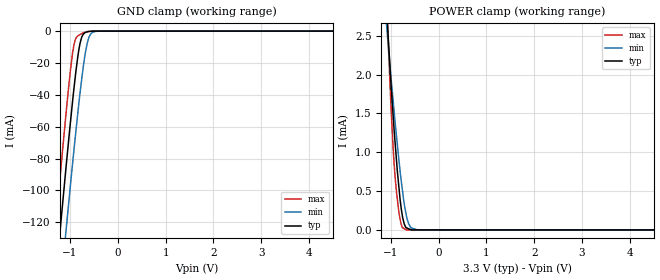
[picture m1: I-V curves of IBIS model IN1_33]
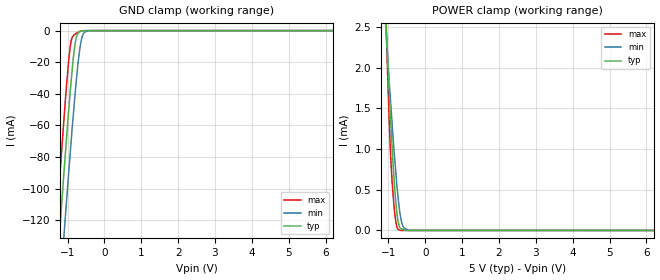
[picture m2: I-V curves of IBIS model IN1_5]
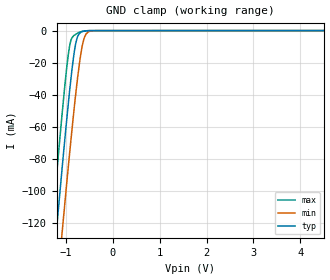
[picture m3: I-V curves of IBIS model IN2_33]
|Texas Instruments Incorporated
|Power Line Communications Analog Front End
| Marketing part#   Digital Voltage Range   Package-type   #pins
|AFE030AIRGZR   2.7 to 5.5 V   VQFN   48
|AFE030AIRGZT   2.7 to 5.5 V   VQFN   48
[IBIS Ver]   4.0
[File name]   afe030.ibs
[File Rev]   1.0
[Date]   11/12/2010
[Source]   Texas Instruments Incorporated.
   Analog-eLab, HPA
   12500 TI Blvd
   Dallas, TX -75243
   For Support e-mail: elab_ibis@list.ti.com
[Notes]   Revision History:
   1.0: 11/12/2010
   - Initial version of the model
   - Initial Model generated from simulations in TISPICED
   - Model names with a trailing _33 contains the model for
   3.3V (3V and 3.6V).
   _ Model names with trailing _5 contains
   the model for 5V (4.5V and 5.5V) operation.
   - Model not matched to measurements
   - C_comp although listed in numerical order of value are
   obtained from varying PVT conditions. For PVT conditions
   for each specific value refer the buffer description under
   respective [Model]. IBIS model user is responsible for using
   appropriate C_comp to simulate for Signal Integrity.
   - Combined nonmonitonicity of OUT_33 and OUT_5 pulldown and
   pullup data is inherent to buffers as seen in simulations
[Disclaimer]
 This product is designed as an aid for customers of Texas Instruments.
 No warranties, either expressed or implied, with respect to this third
 party software (if any) or with respect to its fitness for any
 particular purpose is claimed by Texas Instruments or the author. The
 software (if any) is provided solely on an "as is" basis. The entire
 risk as to its quality and performance is with the customer
[Copyright] (C) Copyright 2009 Texas Instruments Incorporated.
   All rights reserved.
|   AFE031
[Component]   AFE031
[Manufacturer] TI
[Package]   | 48 QFN - RGZ package
| variable   typ   min   max
R_pkg  4.37953E-02   3.97800E-02   4.78600E-02
L_pkg  1.49490E+00nH 1.30880E+00nH 1.70496E+00nH
C_pkg  3.20541E-01pF 3.01690E-01pF 3.38680E-01pF
|-------------------------PIN------------------------------------------------
[Pin] signal_name  model_name  R_pin  L_pin C_pin
1  DGnd   GND   0.04794  1.70441nH  0.32378pF
2  DVdd   POWER  0.04526  1.58988nH  0.33894pF
3  SCLK   IN1   0.04305  1.48606nH  0.32786pF
4  DIN   IN1   0.04124  1.40172nH  0.31704pF
5  DOUT   OUT1   0.04012  1.34655nH  0.30872pF
6  CS   IN1   0.03982  1.32719nH  0.30169pF
7  DAC   IN1   0.04021  1.33885nH  0.30263pF
8  SD   IN1   0.04128  1.38204nH  0.30973pF
9  INT   OUT2   0.04165  1.41439nH  0.31629pF
10 TSense   TERM   0.04363  1.50387nH  0.32778pF
11 AVdd1   POWER  0.04489  1.57822nH  0.33524pF
12 AGnd1   GND   0.04663  1.66363nH  0.31950pF
13 Tx_PGA_In   TERM   0.04786  1.70496nH  0.31944pF
14 Tx_PGA_Out   TERM   0.04650  1.63128nH  0.33542pF
15 Tx_F_In1   TERM   0.04547  1.56285nH  0.32756pF
16 Tx_F_In2   TERM   0.04465  1.50749nH  0.31973pF
17 Tx_F_Out   TERM   0.04404  1.46688nH  0.31329pF
18 PA_In   TERM   0.04373  1.44633nH  0.30627pF
19 C1   TERM   0.04363  1.44263nH  0.30600pF
20 Rx_PGA2_Out  TERM   0.04374  1.45568nH  0.31243pF
21 Rx_PGA2_In   TERM   0.04415  1.48905nH  0.31836pF
22 Rx_F_Out   TERM   0.04479  1.53774nH  0.32624pF
23 Rx_C2   TERM   0.04597  1.60959nH  0.33499pF
24 Rx_C1   TERM   0.04761  1.69090nH  0.31944pF
25 Rx_F_In   TERM   0.04666  1.64938nH  0.32310pF
26 Rx_PGA1_Out  TERM   0.04436  1.54523nH  0.33868pF
27 Rx_PGA1_In   TERM   0.04253  1.45348nH  0.32802pF
28 C2   TERM   0.04110  1.38100nH  0.31750pF
29 AGnd2   GND   0.04027  1.33462nH  0.30931pF
30 AVdd2   POWER  0.03989  1.31213nH  0.30236pF
31 E_Rx_Out   TERM   0.03978  1.30880nH  0.30230pF
32 E_Rx_In   TERM   0.04003  1.32739nH  0.30911pF
33 E_Tx_Out   OUT1   0.04080  1.37171nH  0.31662pF
34 E_Tx_In   IN2   0.04200  1.43702nH  0.32606pF
35 E_Tx_Clk   IN2   0.04357  1.52060nH  0.33618pF
36 ZC_Out2   TERM   0.04571  1.61986nH  0.32130pF
37 ZC_Out1   TERM   0.04717  1.66751nH  0.32302pF
38 ZC_In2   IN3   0.04609  1.60204nH  0.33837pF
39 ZC_In1   IN3   0.04599  1.56391nH  0.33217pF
40 PA_Gnd2   GND   0.04479  1.49878nH  0.32458pF
41 PA_Gnd1   GND   0.04400  1.45436nH  0.32078pF
42 PA_Out2   TERM   0.04316  1.41904nH  0.31296pF
43 PA_Out1   TERM   0.04316  1.41958nH  0.31068pF
44 PA_Vs2   TERM   0.04358  1.44390nH  0.31762pF
45 PA_Vs1   TERM   0.04427  1.48688nH  0.32403pF
46 PA_Iset   TERM   0.04563  1.55774nH  0.33228pF
47 Tx_Flag   OUT2   0.04599  1.60396nH  0.33861pF
48 Rx_Flag   OUT2   0.04709  1.67076nH  0.32210pF
|   Model Selectors
[Model Selector]  IN1
IN1_33  3.3V digital input
IN1_5   5V digital input
|NOTES   Model IN1 split into two Models IN1_33 and IN1_5
|   to accomodate vast voltage range of 2.7V - 5.5V
|   IN1_33 operates in voltage range of 3 - 3.3 - 3.6
|   IN1_5 operates in voltage range of 4.5 - 5 - 5.5
|   The max pin frequency for Model IN1 is 20MHz.Also the
|   voltage range and frequency is referenced with datasheet.
[Model Selector]  IN2
IN2_33  3.3V digital input
IN2_5   5V digital input
|NOTES   Model IN2 split into two Models IN2_33 and IN2_5
|   to accomodate vast voltage range of 2.7V - 5.5V
|   IN2_33 operates in voltage range of 3 - 3.3 - 3.6
|   IN2_5 operates in voltage range of 4.5 - 5 - 5.5
|   The max pin frequency for Model IN2 is 20MHz.Also the
|   voltage range and frequency is referenced with datasheet.
[Model Selector]  IN3
IN3_33  3.3V digital input
IN3_5   5V digital input
|NOTES   Model IN1 split into two Models IN3_33 and IN3_5
|   to accomodate vast voltage range of 2.7V - 5.5V
|   IN3_33 operates in voltage range of 3 - 3.3 - 3.6
|   IN3_5 operates in voltage range of 4.5 - 5 - 5.5
|   The max pin frequency for Model IN3 is 20MHz.Also the
|   voltage range and frequency is referenced with datasheet.
[Model Selector]  OUT1
OUT1_33 3.3V digital tri-state output
OUT1_5  5V digital tri-state output
|NOTES   Model OUT1 split into two Models OUT1_33 and OUT1_5
|   to accomodate vast voltage range of 2.7V - 5.5V
|   OUT1_33 operates in voltage range of 3 - 3.3 - 3.6
|   OUT1_5 operates in voltage range of 4.5 - 5 - 5.5
|   The max pin frequency for Model OUT1 is 20MHz.Also the
|   voltage range and frequency is referenced with datasheet.
[Model Selector]  OUT2
OUT2_33 3.3V digital open drain output
OUT2_5  5V digital open drain output
|   TERM Model
[Model] TERM
Model_type Terminator
C_comp   1e-20   1e-20   1e-20
| variable   typ   min   max
[Voltage Range]   3.3V   2.0V   5.5V
[POWER Clamp Reference]  3.3V   2.0V   5.5V
[GND Clamp Reference]   0.0V   0.0V   0.0V
|Operating Temperature
[Temperature Range]   27   85   -40
| Models and submodels in the file (11): IN1_33 (Input), IN1_5 (Input), IN2_33 (Input), IN2_5 (Input), IN3_33 (Input), IN3_5 (Input), OUT1_33 (3-state), OUT1_5 (3-state), OUT2_33 (Open_drain), OUT2_5 (Open_drain), TERM (Terminator)
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|NOTES   Model OUT1 split into two Models OUT2_33 and OUT2_5
|   to accomodate vast voltage range of 2.7V - 5.5V
|   OUT2_33 operates in voltage range of 3 - 3.3 - 3.6
|   OUT2_5 operates in voltage range of 4.5 - 5 - 5.5
|   The max pin frequency for Model OUT2 is 20MHz.Also the
|   voltage range and frequency is referenced with datasheet.
|   IN1 3.3V Model
[Model]  IN1_33
Model_type Input
Vinl = 0.99
Vinh = 2.31
|   typ   min   max
|   (nom PVT)   (Fast PVT)   (slow PVT)
C_comp   9.6998920e-13  8.1243570e-13  1.1847970e-12
| Where   nom PVT is  Nominal Process, 3.3V, 52C
|   Fast PVT is Strong Process, 3.6V, -40C
|   Slow PVT is Weak Process, 3.0V, 150C
[Voltage Range]   3.3   3   3.6
[Temperature Range]   52   150   -40
[Power Clamp Reference]   3.3   3   3.6
[GND Clamp Reference]   0   0   0
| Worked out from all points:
|   GND clamp passes 1 mA (typ) near -0.68 V on its own axis
|   POWER clamp passes 1 mA (typ) near -0.90 V on its own axis
[GND Clamp]
|   Voltage   I(typ)   I(min)   I(max)
-3.3V     -845.2mA   -871.9mA   -825.8mA
-1.327V   -164.8mA   -203.7mA   -132mA
-1.297V   -154.8mA   -193.9mA   -121.8mA
-1.212V   -126.8mA   -166.2mA   -93.23mA
-1.081V   -84.67mA   -124.5mA   -50.93mA
-943.3mV  -43.27mA   -82.32mA   -13.27mA
-890.9mV  -29.03mA   -66.76mA   -5.56mA
-811.9mV  -11.17mA   -44.55mA   -2.543mA
-725.4mV  -2.138mA   -23.09mA   -1.128mA
-608.4mV  -245.7uA   -4.377mA   -225.9uA
-470.4mV  -22.24uA   -216.1uA   -26.59uA
6.6V      0A         0A         0A
[POWER Clamp]
|   Voltage   I(typ)   I(min)   I(max)
-3.3V     33.39mA    26.31mA    43mA
-1.096V   2.938mA    2.674mA    3.053mA
-1.056V   2.482mA    2.38mA     2.435mA
-993.8mV  1.841mA    1.936mA    1.545mA
-952.9mV  1.469mA    1.663mA    1.058mA
-881.5mV  887.3uA    1.2mA      480.9uA
-782.6mV  271.6uA    629.5uA    71.73uA
-720.4mV  76.82uA    335.4uA    17.06uA
-675.1mV  27.73uA    182.6uA    953.7nA
-581.7mV  3.442uA    29.55uA    941.4nA
-447.9mV  766.7nA    952.9nA    923.9nA
6.6V      0A         0A         0A
|   IN1 5V Model
[Model]  IN1_5
Model_type Input
Vinl = 1.5
Vinh = 3.5
|   typ   min   max
|   (nom PVT)   (Fast PVT)   (slow PVT)
C_comp   8.5997880e-13  7.5144900e-13  1.0683370e-12
| Where   nom PVT is  Nominal Process, 5V, 52C
|   Fast PVT is Strong Process, 5.5V, -40C
|   Slow PVT is Weak Process, 4.5V, 150C
[Voltage Range]   5   4.5   5.5
[Temperature Range]   52   150   -40
[Power Clamp Reference]   5   4.5   5.5
[GND Clamp Reference]   0   0   0
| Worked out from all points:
|   GND clamp passes 1 mA (typ) near -0.68 V on its own axis
|   POWER clamp passes 1 mA (typ) near -0.90 V on its own axis
[GND Clamp]
|   Voltage   I(typ)   I(min)   I(max)
-5V       -1.441A    -1.459A    -1.431A
-1.361V   -176.2mA   -215mA     -143.8mA
-1.301V   -156.2mA   -195.1mA   -123.2mA
-1.216V   -128.3mA   -167.9mA   -94.91mA
-1.09V    -87.54mA   -127.5mA   -53.71mA
-931.4mV  -39.98mA   -78.88mA   -10.97mA
-877.1mV  -25.63mA   -62.76mA   -4.569mA
-784.8mV  -6.975mA   -37.46mA   -2.075mA
-652.4mV  -582.8uA   -9.454mA   -390.7uA
-565.6mV  -153.3uA   -1.796mA   -133.3uA
-367.7mV  -15.3uA    -17.87uA   -22.62uA
10V       0A         0A         0A
[POWER Clamp]
|   Voltage   I(typ)   I(min)   I(max)
-5V       57.59mA    45.47mA    74.5mA
-1.093V   2.913mA    2.651mA    3.018mA
-1.05V    2.422mA    2.343mA    2.349mA
-964.4mV  1.569mA    1.74mA     1.184mA
-900.3mV  1.027mA    1.321mA    601.4uA
-820.1mV  466.2uA    835.9uA    181.4uA
-772.2mV  231.8uA    568uA      47.83uA
-732mV    102uA      381.9uA    9.875uA
-674.8mV  27.86uA    180.2uA    1.228uA
-624.4mV  15.93uA    74.62uA    844.3nA
-434.7mV  519.2nA    664.6nA    829.2nA
10V       0A         0A         0A
|   IN2 3.3V Model
[Model]  IN2_33
Model_type Input
Vinl = 0.99
Vinh = 2.31
|   typ   min   max
|   (nom PVT)   (Fast PVT)   (slow PVT)
C_comp   1.1609210e-12  9.3466370e-13  1.3931720e-12
| Where   nom PVT is  Nominal Process, 3.3V, 52C
|   Fast PVT is Strong Process, 3.6V, -40C
|   Slow PVT is Weak Process, 3.0V, 150C
[Voltage Range]   3.3   3   3.6
[Temperature Range]   52   150   -40
[Power Clamp Reference]   3.3   3   3.6
[GND Clamp Reference]   0   0   0
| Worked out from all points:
|   GND clamp passes 1 mA (typ) near -0.68 V on its own axis
[GND Clamp]
|   Voltage   I(typ)   I(min)   I(max)
-3.3V     -852.2mA   -879.7mA   -831.8mA
-1.336V   -169.6mA   -208.8mA   -136.5mA
-1.296V   -156.2mA   -195.7mA   -123mA
-1.2V     -124.2mA   -164mA     -90.45mA
-1.076V   -84.27mA   -124.4mA   -50.45mA
-939.8mV  -42.96mA   -82.27mA   -13.09mA
-890.9mV  -29.61mA   -67.58mA   -5.935mA
-829.7mV  -15mA      -50.22mA   -3.078mA
-732.3mV  -2.751mA   -25.3mA    -1.293mA
-611.7mV  -347.8uA   -4.891mA   -291.2uA
-463.8mV  -21.56uA   -243.4uA   -27.43uA
6.6V      0A         0A         0A
[POWER Clamp]
|   SCR cell for ESD function. Effects occurr above VDD x 2
|   Voltage   I(typ)   I(min)   I(max)
-3.3V     0A         0A         0A
0V        0A         0A         0A
6.6V      0A         0A         0A
